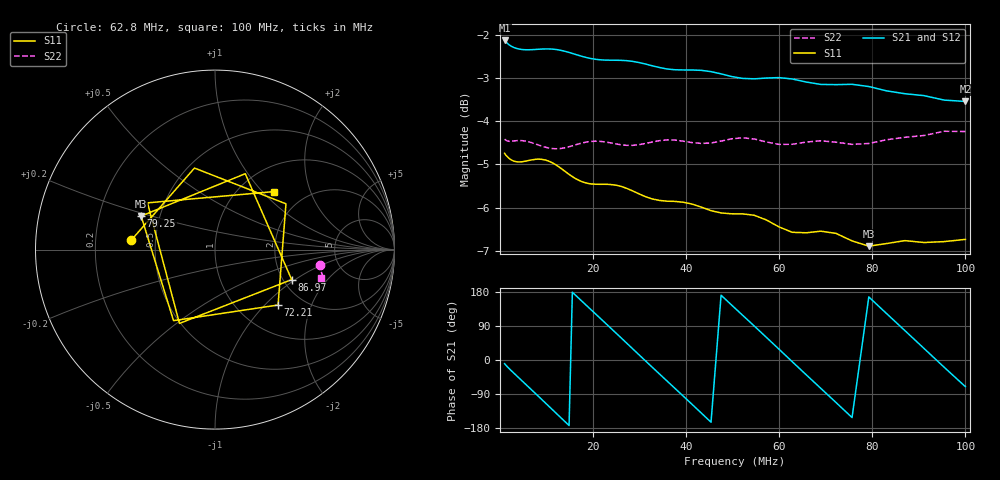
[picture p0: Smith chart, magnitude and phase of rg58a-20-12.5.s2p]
! ListType=Log
!!RG-58A/U 20' SWR=4 L=12.5
# MHZ S RI R 50
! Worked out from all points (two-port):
!   100 points, 1 MHz to 100 MHz, reference 50 ohm
!   highest |S21| = -2.12 dB at 1 MHz (marker M1); lowest = -3.5 dB at 100 MHz (marker M2)
!   |S21| within 3 dB of the highest: start of sweep to end of sweep
!   lowest |S11| = -6.9 dB at 79.25 MHz (marker M3), VSWR 2.65, Z = 19.6 + j9.22 ohm
!   |S11| at or under -10 dB: nowhere
!   |S22| runs from -4.6 to -4.2 dB; largest |S21 - S12| = 0.003
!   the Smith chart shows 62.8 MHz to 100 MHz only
!   S11 on the Smith chart (normalised r, x): 62.8 MHz: 0.36, +0.05; 72.21 MHz: 1.51, -1.20; 79.25 MHz: 0.39, +0.18; 86.97 MHz: 2.22, -0.94; 100 MHz: 1.42, +1.16
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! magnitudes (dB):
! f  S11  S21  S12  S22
! 1 MHz  -4.7  -2.1  -2.1  -4.4
! 3.511 MHz  -4.9  -2.3  -2.3  -4.4
! 10.24 MHz  -4.9  -2.3  -2.3  -4.6
! 13.53 MHz  -5.1  -2.4  -2.4  -4.6
! 17.89 MHz  -5.4  -2.5  -2.5  -4.5
! 21.54 MHz  -5.5  -2.6  -2.6  -4.5
! 25.95 MHz  -5.5  -2.6  -2.6  -4.5
! 34.3 MHz  -5.8  -2.8  -2.7  -4.4
! 39.44 MHz  -5.9  -2.8  -2.8  -4.5
! 43.29 MHz  -6.0  -2.8  -2.8  -4.5
! 47.51 MHz  -6.1  -2.9  -2.9  -4.5
! 52.14 MHz  -6.1  -3.0  -3.0  -4.4
! 54.62 MHz  -6.2  -3.0  -3.0  -4.4
! 59.95 MHz  -6.4  -3.0  -3.0  -4.5
! 62.8 MHz  -6.6  -3.0  -3.0  -4.5
! 68.93 MHz  -6.5  -3.1  -3.1  -4.5
! 72.21 MHz  -6.6  -3.1  -3.1  -4.5
! 79.25 MHz  -6.9  -3.2  -3.2  -4.5
! 86.97 MHz  -6.8  -3.4  -3.3  -4.4
! 91.12 MHz  -6.8  -3.4  -3.4  -4.3
! 95.45 MHz  -6.8  -3.5  -3.5  -4.2
! 100 MHz  -6.7  -3.5  -3.6  -4.2
